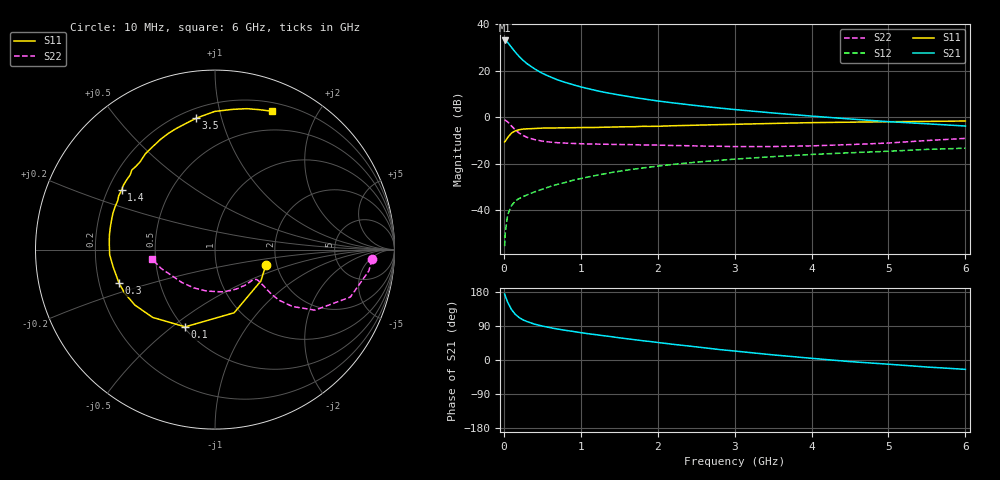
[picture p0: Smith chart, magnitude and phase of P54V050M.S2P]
! SIEMENS Small Signal Semiconductors
! BFP183
! Si NPN RF Bipolar Junction Transistor in SOT143
! VCE = 4 V  IC = 50 mA
! Common Emitter S-Parameters:  March  1996
# GHz  S  MA  R  50
!  f  S11  S21  S12  S22
! GHz  MAG  ANG  MAG  ANG  MAG  ANG  MAG  ANG
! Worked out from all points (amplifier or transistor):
!   36 points, 10 MHz to 6 GHz, reference 50 ohm
!   highest |S21| = 33.1 dB at 10 MHz (marker M1)
!   |S21| within 3 dB of that: start of sweep to 100.5 MHz
!   unconditionally stable (mu >= 1): start of sweep to 14.25 MHz; 379.2 MHz to end of sweep
!   at 250 MHz: K = 0.81, MSG = 29.3 dB, |S12| = -34.1 dB
!   at 1.4 GHz: K = 1.32, MAG = 13.6 dB, |S12| = -23.7 dB
!   at 6 GHz: K = 1.05, MAG = 3.4 dB, |S12| = -13.3 dB
!   S11 on the Smith chart (normalised r, x): 10 MHz: 1.75, -0.33; 100 MHz: 0.51, -0.56; 300 MHz: 0.28, -0.16; 1.4 GHz: 0.26, +0.27; 3.5 GHz: 0.26, +0.83; 6 GHz: 0.29, +1.46
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0.01  0.2958 -16.8  45.01 174.0  0.0017 74.8  0.8773 -3.6
0.02  0.3098 -34.3  44.67 168.5  0.0035 79.3  0.8651 -7.9
0.05  0.3677 -73.1  40.84 152.4  0.0081 70.8  0.7994 -19.3
0.1  0.4614 -111.1  31.95 133.0  0.0127 56.2  0.6513 -31.2
0.15  0.5132 -132.6  25.15 120.2  0.016 52.0  0.5357 -36.3
0.2  0.5429 -145.3  20.3 111.9  0.018 50.7  0.4587 -38.2
0.25  0.5587 -154.2  16.82 105.9  0.0197 51.5  0.4085 -38.4
0.3  0.5663 -160.7  14.32 101.6  0.0215 52.9  0.3728 -37.7
0.4  0.5756 -170.3  11.02 94.6  0.025 54.9  0.332 -36.6
0.5  0.5876 -177.2  8.856 89.6  0.0285 55.9  0.3086 -35.9
0.6  0.5897 177.1  7.473 85.4  0.0325 58.2  0.2942 -35.6
0.7  0.5938 172.3  6.385 81.7  0.0364 60.0  0.285 -35.8
0.8  0.5961 168.2  5.636 78.3  0.0398 60.5  0.2797 -36.5
1.1  0.6056 156.9  4.127 69.2  0.0526 60.8  0.2679 -40.0
1.4  0.6174 147.4  3.242 61.5  0.0652 59.6  0.2626 -45.1
1.8  0.6413 136.3  2.519 51.0  0.0815 57.0  0.2548 -53.3
2.2  0.6603 125.9  2.048 41.4  0.0974 53.4  0.2482 -62.8
2.8  0.6978 111.8  1.59 27.6  0.1193 47.5  0.239 -79.6
3.5  0.7399 98.1  1.242 13.5  0.1432 41.0  0.2357 -101.7
4.5  0.7873 82.9  0.923 -4.2  0.1732 31.1  0.2599 -135.1
5.5  0.8185 72.2  0.727 -18.5  0.2045 22.6  0.3176 -160.6
6  0.8341 67.5  0.651 -24.7  0.2173 17.7  0.3532 -171.3
